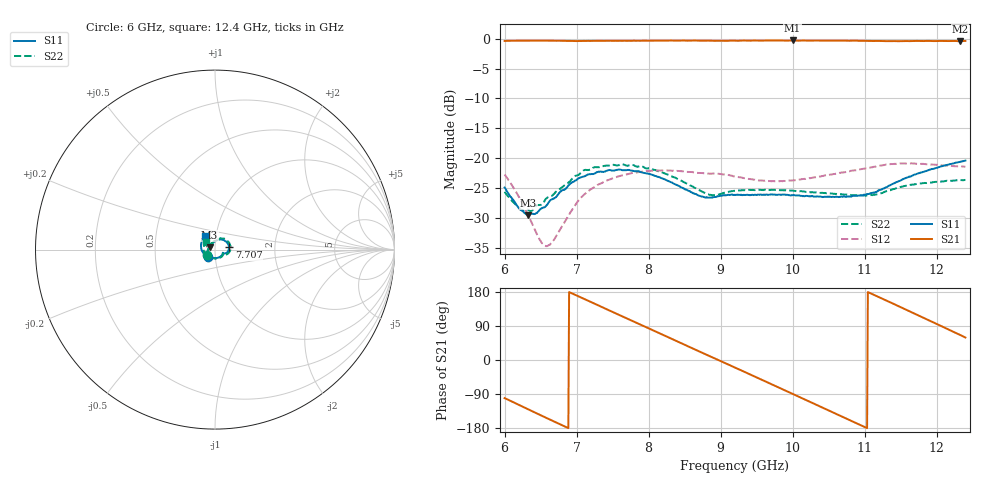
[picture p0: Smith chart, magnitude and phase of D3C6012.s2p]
! 11/4/2020 3:15:29 PM
! C:\USERS\DITOM\DESKTOP\SINGLE JUNCTION ISOLATOR DATA\6.0 - 12.4 GHZ (D3I6012).S2P
! CHANNEL.1
! TR.MEASUREMENT
! CORRECTED.DATA
# GHZ S RI R 50.0
! FREQ.GHZ  S11RE  S11IM  S21RE  S21IM  S12RE  S12IM  S22RE  S22IM
!; PortSelection: Port_12
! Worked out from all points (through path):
!   601 points, 6 GHz to 12.4 GHz, reference 50 ohm
!   highest |S21| = -0.30 dB at 10 GHz (marker M1); lowest = -0.4 dB at 12.33 GHz (marker M2)
!   lowest |S11| = -29.5 dB at 6.331 GHz (marker M3), VSWR 1.07, Z = 47 + j1.27 ohm
!   |S11| at or under -10 dB: start of sweep to end of sweep
!   |S22| runs from -28.8 to -21.0 dB; largest |S21 - S12| = 1
!   S11 on the Smith chart (normalised r, x): 6 GHz: 0.92, -0.07; 7.707 GHz: 1.17, +0.03; 12.4 GHz: 0.88, +0.14
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6  -0.0402 -0.0404  -0.1761 -0.9411  -0.0341 0.0646  -0.0423 -0.0309
6.330667  -0.0305 0.0135  -0.6239 -0.7318  -0.00407 0.0329  -0.0306 0.0207
6.597333  -0.00774 0.0406  -0.8668 -0.4173  -0.011 0.0149  -0.00666 0.0465
6.810667  0.0119 0.0529  -0.9529 -0.1111  -0.0231 0.0155  0.0136 0.0562
7.066667  0.0419 0.0554  -0.9212 0.2555  -0.0318 0.0349  0.0453 0.0613
7.376  0.0664 0.0387  -0.7071 0.6462  -0.01 0.0623  0.0744 0.0433
7.706667  0.0787 0.0132  -0.3096 0.9089  0.0349 0.0646  0.0855 0.0132
8.144  0.0678 -0.0154  0.3107 0.9124  0.0778 0.0128  0.075 -0.0195
8.421333  0.0543 -0.0218  0.6537 0.7068  0.0706 -0.0335  0.0598 -0.0286
8.677333  0.0446 -0.0208  0.8739 0.4043  0.0394 -0.0644  0.0473 -0.0284
8.954667  0.0446 -0.0179  0.9604 0.0191  -0.00869 -0.0736  0.0443 -0.022
9.2  0.0435 -0.0231  0.9029 -0.3315  -0.0495 -0.05  0.0464 -0.0265
9.637333  0.037 -0.0332  0.5131 -0.8169  -0.0595 0.0257  0.0393 -0.0373
10  0.0255 -0.0419  0.0101 -0.966  -0.0104 0.0644  0.0289 -0.0452
10.26667  0.0139 -0.0463  -0.3687 -0.8899  0.0357 0.0584  0.0185 -0.0485
10.55467  -0.000468 -0.0475  -0.7139 -0.6482  0.0701 0.0215  0.00594 -0.0502
10.84267  -0.0165 -0.0455  -0.921 -0.2828  0.0736 -0.0289  -0.00677 -0.0487
11.07733  -0.0295 -0.0415  -0.9562 0.0612  0.053 -0.0645  -0.0167 -0.0459
11.344  -0.048 -0.0345  -0.853 0.4284  0.01 -0.0886  -0.0309 -0.0442
11.87733  -0.0775 0.0149  -0.268 0.9198  -0.0727 -0.051  -0.0617 -0.00811
12.32533  -0.0624 0.0694  0.3845 0.8712  -0.0845 0.0131  -0.055 0.0361
12.4  -0.0562 0.0771  0.4883 0.8231  -0.0816 0.0232  -0.0502 0.0426
